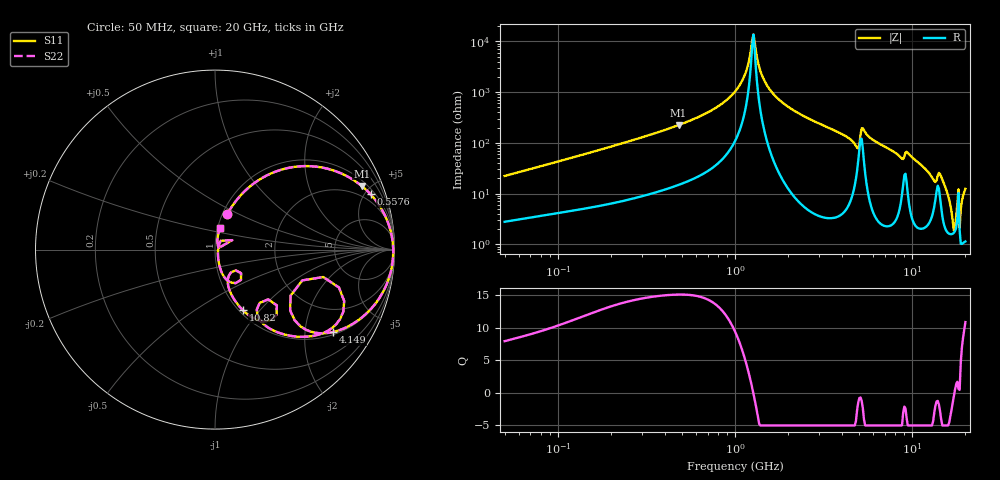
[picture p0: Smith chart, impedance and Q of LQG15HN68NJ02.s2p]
!Murata Part Number: LQG15HN68NJ02
!These Parameters are Measured in Series Mode Connection
!  o--[Z]--o
!Port1  Port2
!  o-------o
!Freq. Start=50[MHz] Stop=20[GHz], 401[Steps]
# Hz S RI R 50
!Freq.(Hz) S11(Real) S11(Imag) S21(Real) S21(Imag) S12(Real) S12(Imag) S22(Real) S22(Imag)
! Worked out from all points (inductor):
!   401 points, 50 MHz to 20 GHz, reference 50 ohm
!   read as one part in series: L = 68.9 nH near 51.52 MHz
!   highest Q = 15.1 at 480 MHz (marker M1), where L = 74 nH
!   self-resonance near 1.252 GHz
!   S11 on the Smith chart (normalised r, x): 50 MHz: 1.06, +0.44; 557.6 MHz: 1.36, +5.48; 4.149 GHz: 1.09, -2.80; 10.82 GHz: 1.04, -0.82; 20 GHz: 1.02, +0.25
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5e7  0.0696 0.1992  0.9304 -0.1992  0.9304 -0.1992  0.0696 0.1992
1.364002e8  0.2672 0.4018  0.7328 -0.4018  0.7328 -0.4018  0.2672 0.4018
3.721004e8  0.7165 0.4184  0.2835 -0.4184  0.2835 -0.4184  0.7165 0.4184
4.800071e8  0.8179 0.3542  0.1821 -0.3542  0.1821 -0.3542  0.8179 0.3542
5.575697e8  0.8672 0.3078  0.1328 -0.3078  0.1328 -0.3078  0.8672 0.3078
1e9  0.9808 0.0942  0.0192 -0.0942  0.0192 -0.0942  0.9808 0.0942
1.144317e9  0.9899 0.0412  0.0101 -0.0412  0.0101 -0.0412  0.9899 0.0412
1.270815e9  0.9928 -0.000668  0.0072 0.000668  0.0072 0.000668  0.9928 -0.000668
1.411297e9  0.9919 -0.043  0.00813 0.043  0.00813 0.043  0.9919 -0.043
1.590961e9  0.986 -0.0919  0.014 0.0919  0.014 0.0919  0.986 -0.0919
2.728004e9  0.8822 -0.3149  0.1178 0.3149  0.1178 0.3149  0.8822 -0.3149
4.149438e9  0.658 -0.459  0.342 0.459  0.342 0.459  0.658 -0.459
4.81993e9  0.4442 -0.3942  0.5558 0.3942  0.5558 0.3942  0.4442 -0.3942
5.117541e9  0.6031 -0.1528  0.3969 0.1528  0.3969 0.1528  0.6031 -0.1528
5.769027e9  0.6129 -0.4604  0.3871 0.4604  0.3871 0.4604  0.6129 -0.4604
7.442007e9  0.3646 -0.4663  0.6354 0.4663  0.6354 0.4663  0.3646 -0.4663
1.082228e10  0.1563 -0.3386  0.8437 0.3386  0.8437 0.3386  0.1563 -0.3386
1.334722e10  0.0759 -0.1467  0.9241 0.1467  0.9241 0.1467  0.0759 -0.1467
1.460232e10  0.0848 -0.1821  0.9152 0.1821  0.9152 0.1821  0.0848 -0.1821
1.597544e10  0.0238 -0.0853  0.9762 0.0853  0.9762 0.0853  0.0238 -0.0853
1.721783e10  0.0165 -0.0075  0.9835 0.0075  0.9835 0.0075  0.0165 -0.0075
2e10  0.0257 0.1187  0.9743 -0.1187  0.9743 -0.1187  0.0257 0.1187
